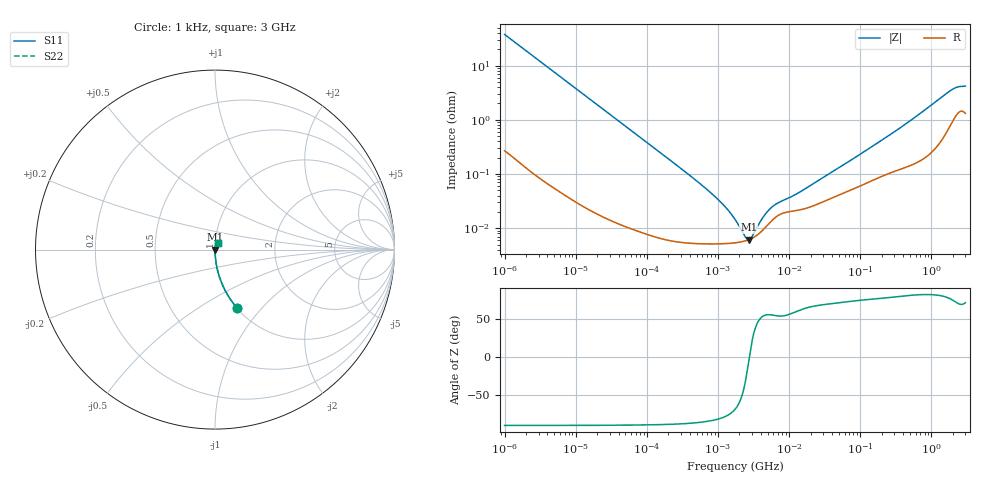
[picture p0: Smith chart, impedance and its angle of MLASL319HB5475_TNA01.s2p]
! MLASL319HB5475_TNA01  S-PARAMETER MODEL  ( Standard Model )
! Model Generated by TAIYO YUDEN Corporation (http://www.ty-top.com)
! Version 1.0
! TAIYO YUDEN Control No. 220601
! Copyright(c) 2009 TAIYO YUDEN CO.,LTD. All Rights Reserved.
! Product Description (link to TY-COMPAS)
! https://ds.yuden.co.jp/TYCOMPAS/or/detail?pn=MLASL319HB5475KTNA01&u=M
! Products Name : Multilayer Ceramic Capacitors
! Characteristics :
!  Capacitance : 4.7 [uF] , Rated Voltage : 10 [V] , TCC : B / X5R
!  Case Size : 3.2 x 1.6 / 0.126 x 0.063 [mm/inch] , Thickness : 0.85 / 0.033 [mm/inch]
!  (Conditions: Temperature = 25 [degC] , DC Bias Voltage = 0 [V])
! External Node Assignments :
!  1  o---| |---o  2
! GND o---------o GND
! Frequency Range : 1kHz  -  3GHz  [ 401 STEP ]
# MHZ S RI R 50
! Freq[MHz].  S11 Real  S11 Imag  S21 Real  S21 Imag  S12 Real  S12 Imag  S22 Real  S22 Imag
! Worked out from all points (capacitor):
!   401 points, 1 kHz to 3 GHz, reference 50 ohm
!   read as one part in series: C = 4.25 uF near 1.077 kHz
!   lowest |Z| = 6.16 mohm at 2.709 MHz (marker M1)
!   series resonance near 2.752 MHz, so ESL is about 790 pH
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0.001  0.1244 -0.3265  0.8756 0.3265  0.8756 0.3265  0.1244 -0.3265
0.001685  0.0485 -0.2113  0.9515 0.2113  0.9515 0.2113  0.0485 -0.2113
0.00306  0.0157 -0.1207  0.9843 0.1207  0.9843 0.1207  0.0157 -0.1207
0.005768  0.00472 -0.065  0.9953 0.065  0.9953 0.065  0.00472 -0.065
0.01216  0.00122 -0.031  0.9988 0.031  0.9988 0.031  0.00122 -0.031
0.147855  7.24e-05 -0.00258  0.9999 0.00258  0.9999 0.00258  7.24e-05 -0.00258
0.43594  5.31e-05 -0.000859  0.9999 0.000859  0.9999 0.000859  5.31e-05 -0.000859
0.821683  5.14e-05 -0.000427  0.9999 0.000427  0.9999 0.000427  5.14e-05 -0.000427
1.285341  5.2e-05 -0.000235  0.9999 0.000235  0.9999 0.000235  5.2e-05 -0.000235
1.732051  5.37e-05 -0.000136  0.9999 0.000136  0.9999 0.000136  5.37e-05 -0.000136
2.087011  5.57e-05 -7.95e-05  0.9999 7.95e-05  0.9999 7.95e-05  5.57e-05 -7.95e-05
2.709407  6.14e-05 -4.42e-06  0.9999 4.42e-06  0.9999 4.42e-06  6.14e-05 -4.42e-06
3.264662  6.94e-05 4.92e-05  0.9999 -4.92e-05  0.9999 -4.92e-05  6.94e-05 4.92e-05
3.517417  7.41e-05 7.08e-05  0.9999 -7.08e-05  0.9999 -7.08e-05  7.41e-05 7.08e-05
4.919932  0.000112 0.000166  0.9999 -0.000166  0.9999 -0.000166  0.000112 0.000166
6.387174  0.000158 0.000223  0.9998 -0.000223  0.9998 -0.000223  0.000158 0.000223
12.49624  0.000211 0.000367  0.9998 -0.000367  0.9998 -0.000367  0.000211 0.000367
21.06097  0.000254 0.000591  0.9997 -0.000591  0.9997 -0.000591  0.000254 0.000591
256.0921  0.00105 0.00508  0.9989 -0.00508  0.9989 -0.00508  0.00105 0.00508
1847.629  0.00889 0.033  0.9911 -0.033  0.9911 -0.033  0.00889 0.033
2310.849  0.014 0.037  0.986 -0.037  0.986 -0.037  0.014 0.037
3000  0.0144 0.0387  0.9856 -0.0387  0.9856 -0.0387  0.0144 0.0387
